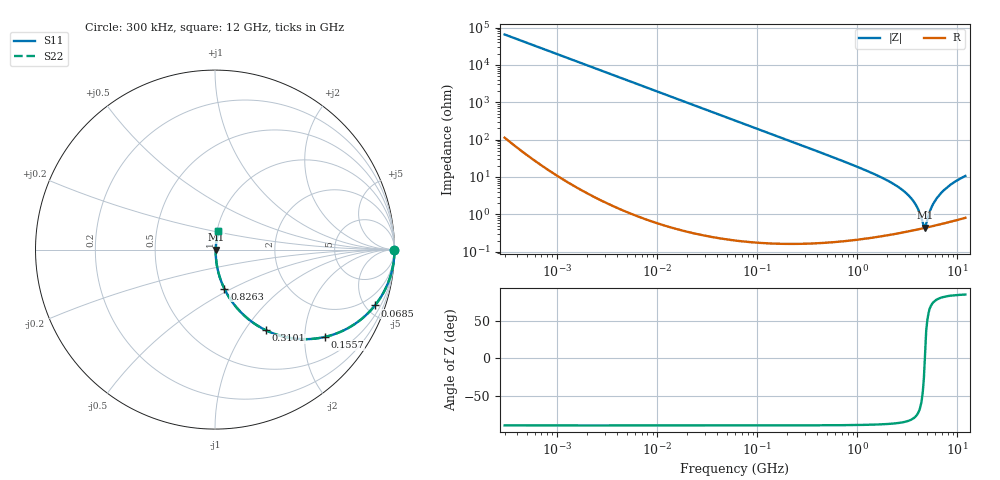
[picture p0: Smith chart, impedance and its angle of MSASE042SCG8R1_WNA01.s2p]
! MSASE042SCG8R1_WNA01  S-PARAMETER MODEL  ( General Type )
! Model Generated by TAIYO YUDEN Corporation (http://www.ty-top.com)
! Version 1.0
! TAIYO YUDEN Control No. 130801
! Copyright(c) 2013 TAIYO YUDEN CO.,LTD. All Rights Reserved.
! Product Description (link to TY-COMPAS)
! https://ds.yuden.co.jp/TYCOMPAS/or/detail?pn=MSASE042SCG8R1BWNA01&u=M
! Products Name : Multilayer Ceramic Capacitors
! Characteristics :
!  Capacitance : 8.1 pF , Rated Voltage : 16V , TCC : CG / C0G
!  Case Size : 0.4 x 0.2 / 0.016 x 0.008 [mm/inch] , Thickness : 0.2 / 0.008 [mm/inch]
!  (Conditions: Temperature = 25 degC , DC Bias Current/Voltage = 0A / 0V)
! External Node Assignments :
!  1  o---| |---o  2
! GND o---------o GND
! Frequency Range : 0.3MHz  -  12000MHz  [ 401 STEP ]
# MHz S RI R 50
! Freq[MHz].  S11 Real  S11 Imag  S21 Real  S21 Imag  S12 Real  S12 Imag  S22 Real  S22 Imag
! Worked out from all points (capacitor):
!   401 points, 300 kHz to 12 GHz, reference 50 ohm
!   read as one part in series: C = 8.11 pF near 316.3 kHz
!   lowest |Z| = 439 mohm at 4.748 GHz (marker M1)
!   series resonance near 4.726 GHz, so ESL is about 140 pH
!   S11 on the Smith chart (normalised r, x): 300 kHz: open; 68.5 MHz: 1.00, -5.73; 155.7 MHz: 1.00, -2.52; 310.1 MHz: 1.00, -1.26; 826.3 MHz: 1.00, -0.46; 12 GHz: 1.02, +0.21
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0.3  1 -0.00153  4.98e-06 0.00153  4.98e-06 0.00153  1 -0.00153
1.769972  0.9999 -0.00902  8.5e-05 0.00902  8.5e-05 0.00902  0.9999 -0.00902
10.44266  0.9972 -0.0531  0.00284 0.0531  0.00284 0.0531  0.9972 -0.0531
27.10171  0.9812 -0.1355  0.0188 0.1355  0.0188 0.1355  0.9812 -0.1355
60  0.9143 -0.2796  0.0857 0.2796  0.0857 0.2796  0.9143 -0.2796
68.49786  0.8911 -0.3111  0.1089 0.3111  0.1089 0.3111  0.8911 -0.3111
101.9188  0.7871 -0.4089  0.2129 0.4089  0.2129 0.4089  0.7871 -0.4089
155.7172  0.6129 -0.4864  0.3871 0.4864  0.3871 0.4864  0.6129 -0.4864
310.0777  0.2846 -0.4499  0.7154 0.4499  0.7154 0.4499  0.2846 -0.4499
353.9943  0.2337 -0.4217  0.7663 0.4217  0.7663 0.4217  0.2337 -0.4217
826.3444  0.052 -0.2178  0.948 0.2178  0.948 0.2178  0.052 -0.2178
2088.533  0.00846 -0.0749  0.9915 0.0749  0.9915 0.0749  0.00846 -0.0749
2795.104  0.00531 -0.0454  0.9947 0.0454  0.9947 0.0454  0.00531 -0.0454
3454.93  0.00432 -0.0264  0.9957 0.0264  0.9957 0.0264  0.00432 -0.0264
3944.255  0.00413 -0.0152  0.9959 0.0152  0.9959 0.0152  0.00413 -0.0152
4502.883  0.00423 -0.00423  0.9958 0.00423  0.9958 0.00423  0.00423 -0.00423
4747.894  0.00434 0.000446  0.9957 -0.000446  0.9957 -0.000446  0.00434 0.000446
4875.354  0.00442 0.0034  0.9956 -0.0034  0.9956 -0.0034  0.00442 0.0034
5565.855  0.00503 0.0156  0.995 -0.0156  0.995 -0.0156  0.00503 0.0156
6524.734  0.00626 0.0311  0.9937 -0.0311  0.9937 -0.0311  0.00626 0.0311
8503.825  0.01 0.0608  0.99 -0.0608  0.99 -0.0608  0.01 0.0608
12000  0.0191 0.1041  0.9809 -0.1041  0.9809 -0.1041  0.0191 0.1041
